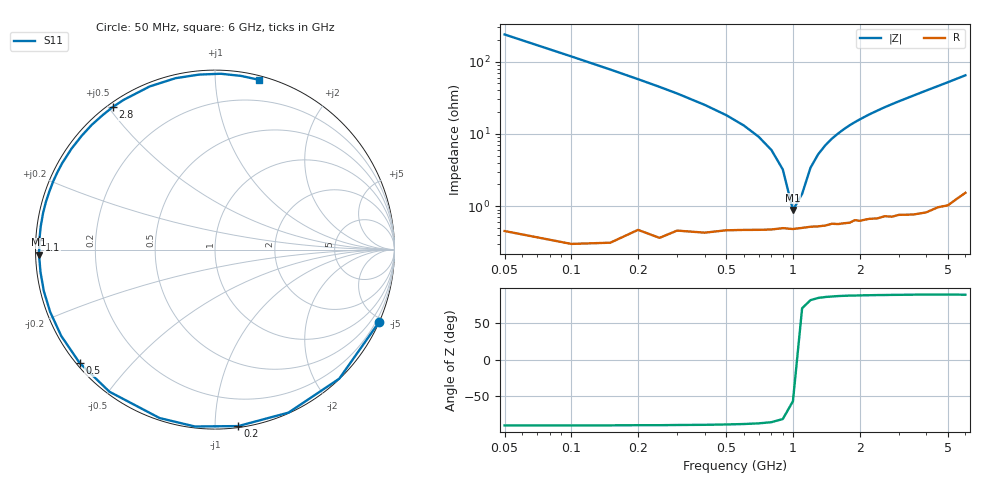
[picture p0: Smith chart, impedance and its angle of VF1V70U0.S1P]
! Infineon Technologies  Discrete & RF Semiconductors
! BBY 58-03
! Si Tuning Diode in SOD323
! VR = 1.75 V
! S-Parameters:  June  1999
# GHz  S  MA  R  50
!  f  S11
! GHz  MAG  ANG
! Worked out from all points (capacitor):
!   34 points, 50 MHz to 6 GHz, reference 50 ohm
!   read as one part to ground: C = 13.4 pF near 50 MHz
!   lowest |Z| = 886 mohm at 1 GHz (marker M1)
!   series resonance near 1.035 GHz, so ESL is about 1.8 nH
!   S11 on the Smith chart (normalised r, x): 50 MHz: 0.01, -4.72; 200 MHz: 0.01, -1.14; 500 MHz: 0.01, -0.36; 1.1 GHz: 0.01, +0.03; 2.8 GHz: 0.01, +0.51; 6 GHz: 0.03, +1.29
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0.05  0.9992 -23.9
0.1  0.9981 -46.1
0.15  0.9963 -65.7
0.2  0.9918 -82.5
0.25  0.9919 -96.5
0.3  0.988 -108.2
0.4  0.9863 -126.6
0.5  0.9837 -140.1
0.6  0.9825 -150.7
0.7  0.9819 -159.3
0.8  0.9813 -166.4
0.9  0.9803 -172.7
1  0.9808 -178.3
1.1  0.9801 176.8
1.3  0.9793 168.1
1.6  0.9784 157.1
1.8  0.9781 150.6
2  0.9773 144.9
2.2  0.9767 139.5
2.4  0.9771 134.6
2.8  0.9776 125.5
3  0.9771 121.3
3.5  0.9791 111.8
4  0.98 103.0
4.5  0.9791 95.2
5  0.9803 88.1
5.5  0.9785 81.5
6  0.9772 75.6
